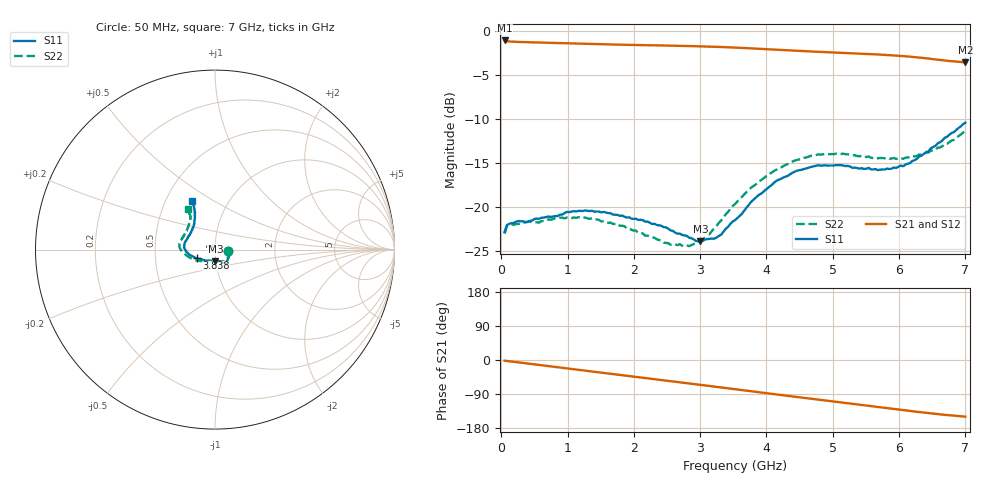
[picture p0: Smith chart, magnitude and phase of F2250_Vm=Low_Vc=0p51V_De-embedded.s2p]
! Integrated Device Technology
! Corporate Headquarters
! 6024 Silver Creek Valley Road
! San Jose, CA 95138  USA
! Phone:  1-408-284-8200
! Toll Free:  1-800-223-1366
! Webpage:  http://www.idt.com/
! Timing and RF Division
! 515 Groton Road, Suite 102
! Westford, MA 01886-6024
! Device:  F2250
! Description: Voltage Variable RF Attenuator
! Frequency:  50.0 -  6000.00 MHz
! Package:  3x3 mm Thin QFN Plastic Package: 16 pin
! Ports:  2 RF, 3 DC
!  Pin  1  = GND
!  Pin  2  = NC
!  Pin  3  = RF1  = Port 1
!  Pin  4  = NC
!  Pin  5  = GND
!  Pin  6  = GND
!  Pin  7  = GND
!  Pin  8  = GND
!  Pin  9  = NC
!  Pin 10  = RF2  = Port 2
!  Pin 11  = NC
!  Pin 12  = GND
!  Pin 13  = GND
!  Pin 14  = VCNTRL
!  Pin 15  = VDD
!  Pin 16  = VMODE
! Vcntrl:  0.510 Volts
! Vmode:  +0.000 Volts
! Vdd:  +3.30  Volts
! Current:  1.130 mA
! Data:  The device was measured on a the F2250 evaluation board which has
!  individual transmission lines to the RF pins.  Data was collected
!  using a calibrated network analyzer.  The evaluation board was
!  de-embedded using a TRL calibration technique.
!  The reference plane is the edge of the package pin.
! Misc:  SN 10
!  Action Tracker AT0258
! Date Measured:  2014-11-26
! Date:  2015-10-15  MJV
! Note:
!  Integrated Device Technology supplies this data as a sample of measured
!  data at the package pin for this product.  Your particular data for this
!  product may vary.
!  Data was taken at 25 degrees C.
!  Integrated Device Technology reserves the right to change this data at anytime.
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# GHz S dB R 50
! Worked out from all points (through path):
!   201 points, 50 MHz to 7 GHz, reference 50 ohm
!   highest |S21| = -1.09 dB at 50 MHz (marker M1); lowest = -3.6 dB at 7 GHz (marker M2)
!   group delay of S21, straight-line fit = 60.1 ps
!   lowest |S11| = -23.8 dB at 3.004 GHz (marker M3), VSWR 1.14, Z = 49.8 - j6.43 ohm
!   |S11| at or under -10 dB: start of sweep to end of sweep
!   |S22| runs from -24.4 to -11.4 dB; largest |S21 - S12| = 0.00043
!   S11 on the Smith chart (normalised r, x): 50 MHz: 1.15, -0.02; 3.838 GHz: 0.81, -0.08; 7 GHz: 0.67, +0.41
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0.05  -22.79 -7.6  -1.09 -1.8  -1.09 -1.8  -22.98 -8.5
0.08475  -22.01 -7.6  -1.17 -2.5  -1.17 -2.5  -22.15 -7.9
0.15425  -21.80 -9.7  -1.22 -4.0  -1.22 -4.0  -21.93 -9.7
0.71025  -21.04 -32.7  -1.36 -16.2  -1.36 -16.2  -21.37 -35.2
1.2315  -20.42 -49.0  -1.47 -27.4  -1.47 -27.4  -21.19 -55.5
1.75275  -20.85 -55.8  -1.56 -38.5  -1.56 -38.5  -21.85 -64.3
2.37825  -22.05 -57.7  -1.65 -51.8  -1.65 -51.8  -23.70 -70.4
2.7605  -23.18 -69.7  -1.71 -60.2  -1.71 -60.2  -24.40 -87.5
2.93425  -23.81 -80.4  -1.75 -64.0  -1.74 -64.0  -24.16 -100.5
3.00375  -23.84 -87.8  -1.76 -65.6  -1.76 -65.6  -23.75 -106.8
3.247  -23.41 -110.5  -1.82 -71.0  -1.81 -71.0  -22.10 -125.6
3.525  -21.46 -136.1  -1.90 -77.2  -1.90 -77.2  -19.63 -142.7
3.83775  -18.91 -154.4  -2.02 -84.1  -2.01 -84.1  -17.41 -156.9
4.1505  -16.99 -167.1  -2.14 -90.9  -2.14 -90.9  -15.73 -169.0
4.4285  -15.96 -175.4  -2.25 -97.0  -2.25 -97.0  -14.70 -176.5
4.7065  -15.37 177.5  -2.35 -103.0  -2.35 -103.0  -14.16 177.3
5.15825  -15.25 166.6  -2.51 -112.7  -2.51 -112.7  -13.92 167.7
5.85325  -15.66 143.0  -2.76 -127.6  -2.76 -127.6  -14.49 152.2
6.166  -14.99 131.4  -2.93 -134.4  -2.93 -134.5  -14.34 143.2
6.444  -13.64 122.3  -3.14 -140.2  -3.14 -140.3  -13.79 133.8
6.82625  -11.48 116.0  -3.45 -146.9  -3.45 -146.9  -12.36 125.7
7  -10.41 115.1  -3.58 -149.5  -3.58 -149.6  -11.36 124.1
